|   TEXAS INSTRUMENTS INCORPORATED
|   Standard Linear and Logic
|   IBIS Model of SN74LVTH273
|   3.3-V ABT OCTAL D-TYPE FLIP-FLOPS WITH CLEAR
|   SOIC 20-pin (DW), SOP 20-pin (NS)
|   SSOP 20-pin (DB), TSSOP 20-pin (PW)
[IBIS Ver]   3.2
[Comment Char] |_char
[File Name]   sn74lvth273.ibs
[File Rev]   1.2 | a_die
[Date]   11/30/04
[Source]   File originated at Texas Instruments, Inc.
[Notes]   The following is a sample IBIS file for the SN74LVTH273.
   - FILE REV HISTORY
   - 1.2 Re-Release IBIS file on 12/16/04
   - All test data contained in this file are derived from
   actual measurement.
   - The measurement used NS package.
   - We have data across voltage and temperature, but not across
   process.
   - Since this is a BiCMOS process, we have irregular trend for the
   curves at high and low temperatures. This data was taken with
   high temperature for strong case and low for weak case.
   - Due to presence of BUS-HOLD at input, GND-CLAMP curves
   have non-monotonic warnings.
   - As there is no power clamp diode we removed the Pwr Clamp
   table data
   - File created by Nobuhisa Ohtsubo, TIJ SLL Product Engineering.
|*   Property of Texas Instruments Incorporated.  Unauthorized   *
|*   reproduction and/or distribution is strictly prohibited.   *
|*   This product is protected under copyright law.   *
|*   Created 1998, (C) Copyright 1998, Texas Instruments Inc.,   *
|*   All Rights Reserved   *
|*   UNLESS THERE IS A SIGNED, WRITTEN AGREEMENT TO THE   *
|*   CONTRARY, TEXAS INSTRUMENTS ("TI") IS PROVIDING THE SPICE   *
|*   MODELS "AS IS" AND WITHOUT ANY WARRANTY, EXPRESSED OR   *
|*   IMPLIED.  TI assumes no liability for:   *
|*   1) the accuracy of the IBIS models provided to your   *
|*   company;   *
|*   2) the proper functioning of these IBIS models in your   *
|*   design or for any resulting applications; or   *
|*   3) infringement of patents, copyrights or intellectual   *
|*   property rights resulting from your use of these   *
|*   IBIS models.   *
|*   TI provides IBIS Models as a service to our customers.   *
|*   You and your company shall not distribute, sell or give   *
|*   these models to anyone else without prior written   *
|*   permission from TI.   *
|*   TI reserves the right to make changes to our products or   *
|*   to discontinue any semiconductor product or service   *
|*   without notice, and advises our customers to obtain the   *
|*   latest version of relevant information to verify, before   *
|*   placing orders, that the information being relied on is   *
|*   current.   *
|*   Please be aware that your receipt and use of the IBIS   *
|*   information provided shall serve as acceptance of these   *
|*   terms and conditions.  If you do not accept these terms,   *
|*   you should return or destroy the IBIS models and any   *
|*   other accompanying information immediately.   *
|   Component LVTH273_DW
[Component]   LVTH273_DW
[Manufacturer]  Texas Instruments, Inc.
[Package]
|   typ   min   max
R_pkg   0.038   0.033   0.045
L_pkg   5.012nH   4.110nH   6.349nH
C_pkg   0.717pF   0.530pF   0.868pF
[Pin]  signal_name  model_name   R_pin   L_pin   C_pin
1   CLR_BAR   LVTH273_CLR   0.042   6.336nH   0.865pF
2   1Q   LVTH273_OUT   0.043   5.542nH   0.867pF
3   1D   LVTH273_IN   0.034   4.714nH   0.732pF
4   2D   LVTH273_IN   0.034   4.377nH   0.591pF
5   2Q   LVTH273_OUT   0.036   4.130nH   0.533pF
6   3Q   LVTH273_OUT   0.035   4.111nH   0.530pF
7   3D   LVTH273_IN   0.034   4.284nH   0.583pF
8   4D   LVTH273_IN   0.034   4.634nH   0.726pF
9   4Q   LVTH273_OUT   0.040   5.518nH   0.865pF
10   GND   GND   0.043   6.349nH   0.866pF
11   CLK   LVTH273_CLK   0.041   6.281nH   0.861pF
12   5Q   LVTH273_OUT   0.045   5.561nH   0.868pF
13   5D   LVTH273_IN   0.033   4.778nH   0.742pF
14   6D   LVTH273_IN   0.035   4.414nH   0.596pF
15   6Q   LVTH273_OUT   0.035   4.110nH   0.533pF
16   7Q   LVTH273_OUT   0.036   4.130nH   0.533pF
17   7D   LVTH273_IN   0.034   4.377nH   0.591pF
18   8D   LVTH273_IN   0.034   4.714nH   0.731pF
19   8Q   LVTH273_OUT   0.043   5.569nH   0.868pF
20   VCC   POWER   0.042   6.308nH   0.864pF
|   Component LVTH273_NS
[Component]   LVTH273_NS
[Manufacturer]  Texas Instruments, Inc.
[Package]
|   typ   min   max
R_pkg   0.044   0.029   0.058
L_pkg   3.666nH   2.317nH   5.115nH
C_pkg   0.548pF   0.316pF   0.725pF
[Pin]  signal_name  model_name   R_pin   L_pin   C_pin
1   CLR_BAR   LVTH273_CLR   0.058   5.115nH   0.725pF
2   1Q   LVTH273_OUT   0.053   4.591nH   0.724pF
3   1D   LVTH273_IN   0.049   3.754nH   0.572pF
4   2D   LVTH273_IN   0.029   2.549nH   0.388pF
5   2Q   LVTH273_OUT   0.031   2.317nH   0.316pF
6   3Q   LVTH273_OUT   0.031   2.317nH   0.316pF
7   3D   LVTH273_IN   0.029   2.556nH   0.399pF
8   4D   LVTH273_IN   0.049   3.754nH   0.579pF
9   4Q   LVTH273_OUT   0.053   4.591nH   0.724pF
10   GND   GND   0.058   5.115nH   0.725pF
11   CLK   LVTH273_CLK   0.058   5.115nH   0.725pF
12   5Q   LVTH273_OUT   0.053   4.591nH   0.724pF
13   5D   LVTH273_IN   0.049   3.754nH   0.579pF
14   6D   LVTH273_IN   0.029   2.557nH   0.399pF
15   6Q   LVTH273_OUT   0.031   2.317nH   0.316pF
16   7Q   LVTH273_OUT   0.031   2.317nH   0.316pF
17   7D   LVTH273_IN   0.029   2.557nH   0.399pF
18   8D   LVTH273_IN   0.049   3.754nH   0.579pF
19   8Q   LVTH273_OUT   0.053   4.591nH   0.724pF
20   VCC   POWER   0.058   5.115nH   0.725pF
|   Component LVTH273_DB
[Component]   LVTH273_DB
[Manufacturer]  Texas Instruments, Inc.
[Package]
|   typ   min   max
R_pkg   0.040   0.035   0.051
L_pkg   3.495nH   3.035nH   4.314nH
C_pkg   0.420pF   0.346pF   0.502pF
[Pin]  signal_name  model_name   R_pin   L_pin   C_pin
1   CLR_BAR   LVTH273_CLR   0.049   4.310nH   0.502pF
2   1Q   LVTH273_OUT   0.048   3.903nH   0.487pF
3   1D   LVTH273_IN   0.035   3.189nH   0.396pF
4   2D   LVTH273_IN   0.035   3.036nH   0.347pF
5   2Q   LVTH273_OUT   0.035   3.035nH   0.367pF
6   3Q   LVTH273_OUT   0.035   3.035nH   0.367pF
7   3D   LVTH273_IN   0.035   3.036nH   0.347pF
8   4D   LVTH273_IN   0.035   3.189nH   0.397pF
9   4Q   LVTH273_OUT   0.047   3.899nH   0.488pF
10   GND   GND   0.051   4.314nH   0.500pF
11   CLK   LVTH273_CLK   0.051   4.314nH   0.500pF
12   5Q   LVTH273_OUT   0.047   3.899nH   0.488pF
13   5D   LVTH273_IN   0.035   3.189nH   0.397pF
14   6D   LVTH273_IN   0.035   3.036nH   0.346pF
15   6Q   LVTH273_OUT   0.035   3.035nH   0.367pF
16   7Q   LVTH273_OUT   0.035   3.035nH   0.367pF
17   7D   LVTH273_IN   0.035   3.036nH   0.346pF
18   8D   LVTH273_IN   0.035   3.189nH   0.397pF
19   8Q   LVTH273_OUT   0.047   3.899nH   0.488pF
20   VCC   POWER   0.051   4.314nH   0.502pF
|   Component LVTH273_PW
[Component]   LVTH273_PW
[Manufacturer]  Texas Instruments, Inc.
[Package]
|   typ   min   max
R_pkg   0.035   0.024   0.047
L_pkg   2.399nH   1.710nH   3.250nH
C_pkg   0.284pF   0.166pF   0.418pF
[Pin]  signal_name  model_name   R_pin   L_pin   C_pin
1   CLR_BAR   LVTH273_CLR   0.041   3.102nH   0.410pF
2   1Q   LVTH273_OUT   0.040   2.777nH   0.363pF
3   1D   LVTH273_IN   0.029   2.194nH   0.260pF
4   2D   LVTH273_IN   0.025   1.710nH   0.166pF
5   2Q   LVTH273_OUT   0.025   1.740nH   0.191pF
6   3Q   LVTH273_OUT   0.024   1.763nH   0.193pF
7   3D   LVTH273_IN   0.024   1.817nH   0.174pF
8   4D   LVTH273_IN   0.028   2.256nH   0.265pF
9   4Q   LVTH273_OUT   0.045   2.887nH   0.368pF
10   GND   GND   0.047   3.250nH   0.417pF
11   CLK   LVTH273_CLK   0.046   3.244nH   0.418pF
12   5Q   LVTH273_OUT   0.046   2.961nH   0.375pF
13   5D   LVTH273_IN   0.033   2.334nH   0.268pF
14   6D   LVTH273_IN   0.029   1.915nH   0.179pF
15   6Q   LVTH273_OUT   0.031   1.934nH   0.203pF
16   7Q   LVTH273_OUT   0.032   1.917nH   0.201pF
17   7D   LVTH273_IN   0.030   1.833nH   0.173pF
18   8D   LVTH273_IN   0.036   2.324nH   0.268pF
19   8Q   LVTH273_OUT   0.042   2.869nH   0.372pF
20   VCC   POWER   0.042   3.160nH   0.414pF
[Model Selector]   LVTH273_IN
LVTH273_IN_28   2.8-V Vcc Input Model
LVTH273_IN_33   3.3-V Vcc Input Model
[Model Selector]   LVTH273_CLR
LVTH273_CLR_28   2.8-V Vcc Input Model
LVTH273_CLR_33   3.3-V Vcc Input Model
[Model Selector]   LVTH273_CLK
LVTH273_CLK_28   2.8-V Vcc Input Model
LVTH273_CLK_33   3.3-V Vcc Input Model
[Model Selector]   LVTH273_OUT
LVTH273_OUT_28   2.8-V Vcc Output Model
LVTH273_OUT_33   3.3-V Vcc Output Model
| Models and submodels in the file (8): LVTH273_IN_28 (Input), LVTH273_CLR_28 (Input), LVTH273_CLK_28 (Input), LVTH273_OUT_28 (Output), LVTH273_IN_33 (Input), LVTH273_CLR_33 (Input), LVTH273_CLK_33 (Input), LVTH273_OUT_33 (Output)
